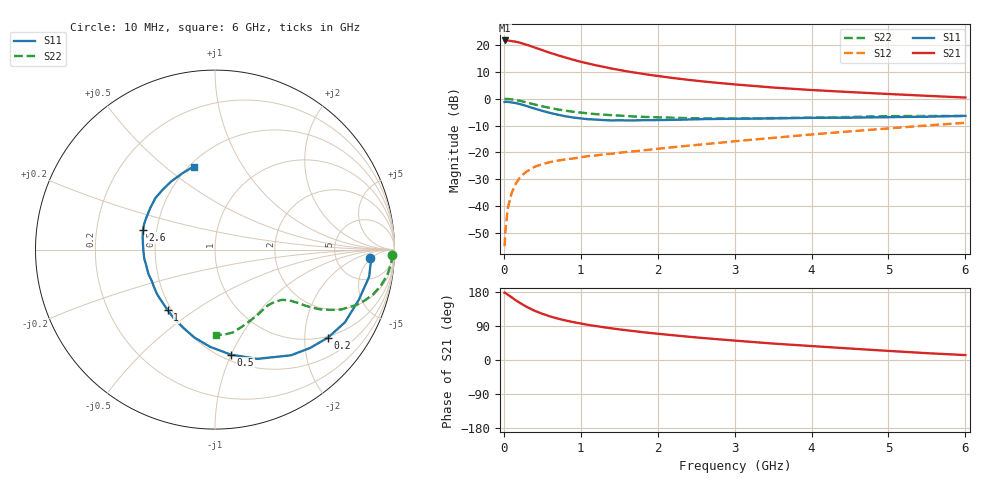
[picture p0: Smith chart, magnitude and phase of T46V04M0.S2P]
! Infineon Technologies  Discrete & RF Semiconductors
! BFR182T
! Si NPN RF Bipolar Junction Transistor in SC75
! VCE = 6 V  IC = 4 mA
! Common Emitter S-Parameters:  October  1999
# GHz  S  MA  R  50
!  f  S11  S21  S12  S22
! GHz  MAG  ANG  MAG  ANG  MAG  ANG  MAG  ANG
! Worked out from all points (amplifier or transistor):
!   36 points, 10 MHz to 6 GHz, reference 50 ohm
!   highest |S21| = 21.6 dB at 10 MHz (marker M1)
!   |S21| within 3 dB of that: start of sweep to 439.5 MHz
!   unconditionally stable (mu >= 1): 1.606 GHz to 4.157 GHz
!   at 250 MHz: K = 0.23, MSG = 24.3 dB, |S12| = -28.2 dB
!   at 1.4 GHz: K = 0.95, MSG = 15.9 dB, |S12| = -20.5 dB
!   at 6 GHz: K = 0.84, MSG = 4.7 dB, |S12| = -9.0 dB
!   S11 on the Smith chart (normalised r, x): 10 MHz: 12, -4; 200 MHz: 0.96, -2.60; 500 MHz: 0.55, -1.00; 1 GHz: 0.48, -0.40; 2.6 GHz: 0.42, +0.11; 6 GHz: 0.53, +0.63
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0.01  0.8657 -3.0  12.09 177.6  0.0018 80.9  0.9851 -1.6
0.02  0.8723 -2.7  12.02 177.1  0.0034 93.3  0.9878 -1.7
0.05  0.872 -10.0  12.04 172.5  0.0089 87.1  0.985 -4.3
0.1  0.8488 -19.2  11.78 165.6  0.0173 81.2  0.9699 -8.5
0.15  0.8297 -29.2  11.48 158.3  0.0254 75.3  0.9451 -12.3
0.2  0.7979 -37.9  11.08 151.7  0.0327 71.6  0.9155 -15.8
0.25  0.7621 -46.0  10.53 145.7  0.0389 67.6  0.8805 -18.8
0.3  0.7252 -54.3  10 139.9  0.0444 63.6  0.8476 -21.3
0.4  0.6529 -68.8  8.957 129.9  0.0539 58.3  0.778 -25.4
0.5  0.5924 -81.3  7.975 122.0  0.0604 55.1  0.7199 -27.8
0.6  0.5423 -92.9  7.126 115.0  0.0659 53.0  0.6711 -29.7
0.7  0.5034 -103.1  6.417 109.4  0.0703 51.5  0.6296 -30.8
0.8  0.4696 -112.3  5.822 104.4  0.074 50.4  0.5975 -31.7
1  0.4286 -127.9  4.85 96.3  0.0812 50.4  0.551 -32.6
1.1  0.4137 -135.9  4.488 92.5  0.0854 50.4  0.5308 -33.4
1.5  0.3949 -159.1  3.42 80.8  0.0983 52.8  0.4835 -35.6
2.2  0.4033 175.1  2.419 65.3  0.1249 56.4  0.4416 -41.7
2.6  0.416 164.7  2.082 57.8  0.1418 58.2  0.4296 -46.1
3.5  0.4288 147.2  1.609 43.4  0.1863 59.8  0.4346 -57.2
4.5  0.4428 131.4  1.324 30.3  0.246 58.5  0.4555 -71.0
5.5  0.4622 113.3  1.128 18.0  0.3166 54.8  0.4765 -83.7
6  0.478 104.5  1.048 13.0  0.355 51.7  0.475 -89.1
